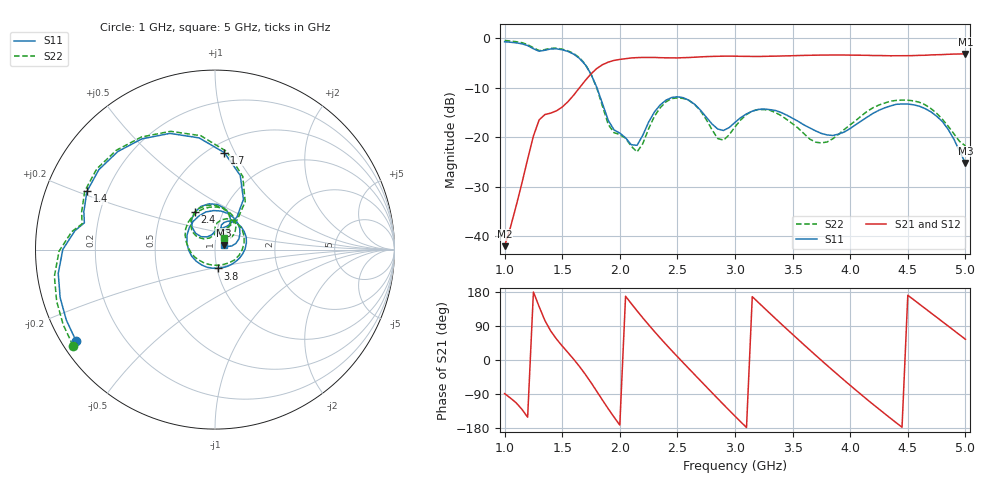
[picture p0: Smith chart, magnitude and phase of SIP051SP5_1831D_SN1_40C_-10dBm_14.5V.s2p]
# GHz  S  dB  R  50
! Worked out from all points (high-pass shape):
!   81 points, 1 GHz to 5 GHz, reference 50 ohm
!   highest |S21| = -3.12 dB at 5 GHz (marker M1); lowest = -42.0 dB at 1 GHz (marker M2)
!   |S21| within 3 dB of the highest: 1.798 GHz to end of sweep
!   lowest |S11| = -25.2 dB at 5 GHz (marker M3), VSWR 1.12, Z = 55.1 + j2.68 ohm
!   |S11| at or under -10 dB: 1.802 GHz to end of sweep
!   |S22| runs from -22.9 to -0.4 dB; largest |S21 - S12| = 0.0021
!   S11 on the Smith chart (normalised r, x): 1 GHz: 0.04, -0.30; 1.4 GHz: 0.13, +0.21; 1.7 GHz: 0.59, +0.91; 2.4 GHz: 0.74, +0.33; 3.8 GHz: 1.01, -0.21; 5 GHz: 1.10, +0.05
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1  -0.66 -146.7  -42.01 -88.7  -42.26 -88.8  -0.40 -145.9
1.25  -2.08 172.3  -19.73 179.4  -19.71 179.5  -1.89 172.9
1.4  -2.12 155.5  -15.10 76.7  -15.09 76.8  -1.99 155.8
1.55  -2.62 123.4  -12.78 19.6  -12.75 19.6  -2.51 123.2
1.7  -5.31 84.5  -8.50 -37.6  -8.52 -37.6  -5.19 83.1
1.85  -13.22 56.0  -5.30 -106.0  -5.29 -106.0  -13.71 53.2
2.05  -20.09 91.2  -4.08 168.2  -4.09 168.2  -20.19 88.3
2.2  -19.56 136.9  -3.83 111.0  -3.84 111.1  -21.26 136.6
2.35  -13.45 127.7  -3.88 58.2  -3.89 58.2  -14.03 133.5
2.4  -12.50 118.3  -3.91 41.5  -3.92 41.4  -12.83 123.2
2.55  -11.97 87.3  -3.88 -7.0  -3.89 -7.0  -12.13 89.7
2.75  -15.89 58.3  -3.67 -70.4  -3.67 -70.4  -16.37 56.1
3  -16.96 75.4  -3.58 -148.1  -3.57 -148.1  -17.88 89.6
3.2  -14.36 50.1  -3.64 152.7  -3.63 152.6  -14.39 58.7
3.4  -14.97 11.6  -3.54 95.5  -3.54 95.6  -15.59 12.8
3.7  -18.70 -53.4  -3.38 12.5  -3.38 12.6  -20.98 -78.4
3.8  -19.51 -81.8  -3.35 -14.4  -3.35 -14.5  -20.93 -115.1
4.05  -17.41 -163.9  -3.38 -79.7  -3.37 -79.8  -16.58 176.6
4.35  -13.65 115.3  -3.50 -153.8  -3.49 -153.8  -12.67 115.8
4.55  -13.42 70.7  -3.46 159.3  -3.45 159.2  -12.62 78.6
4.75  -15.72 31.8  -3.29 112.9  -3.30 112.8  -15.12 48.2
5  -25.19 26.2  -3.12 54.7  -3.11 54.8  -21.73 49.8
